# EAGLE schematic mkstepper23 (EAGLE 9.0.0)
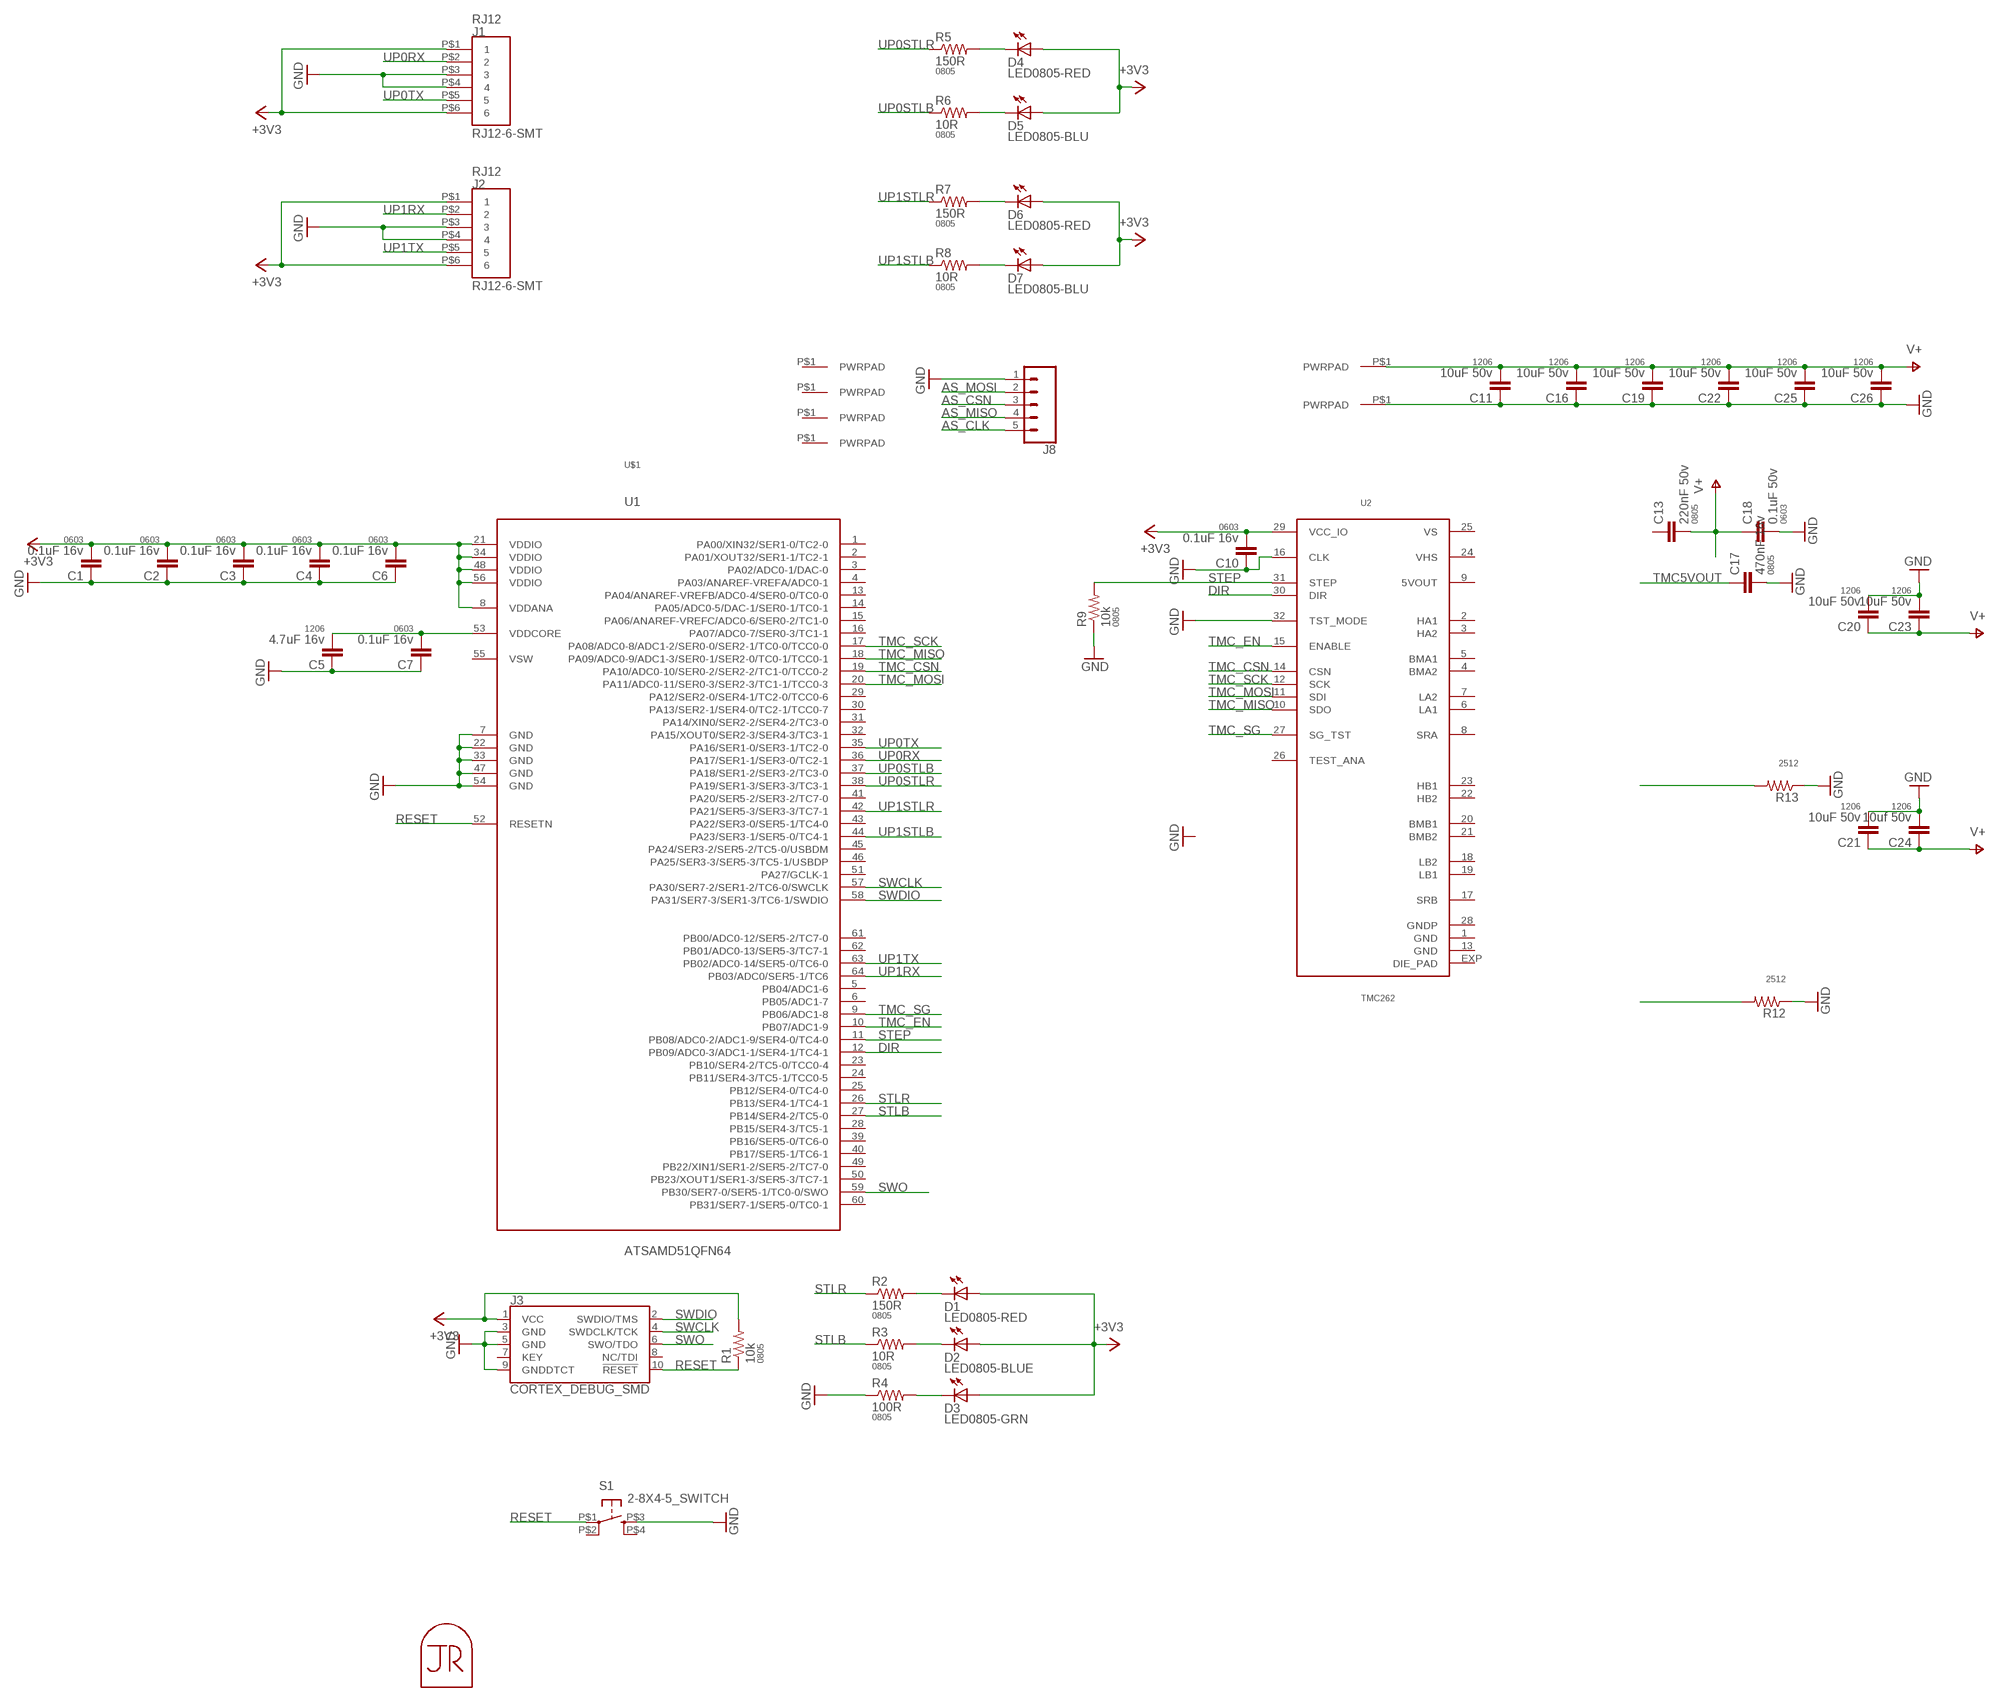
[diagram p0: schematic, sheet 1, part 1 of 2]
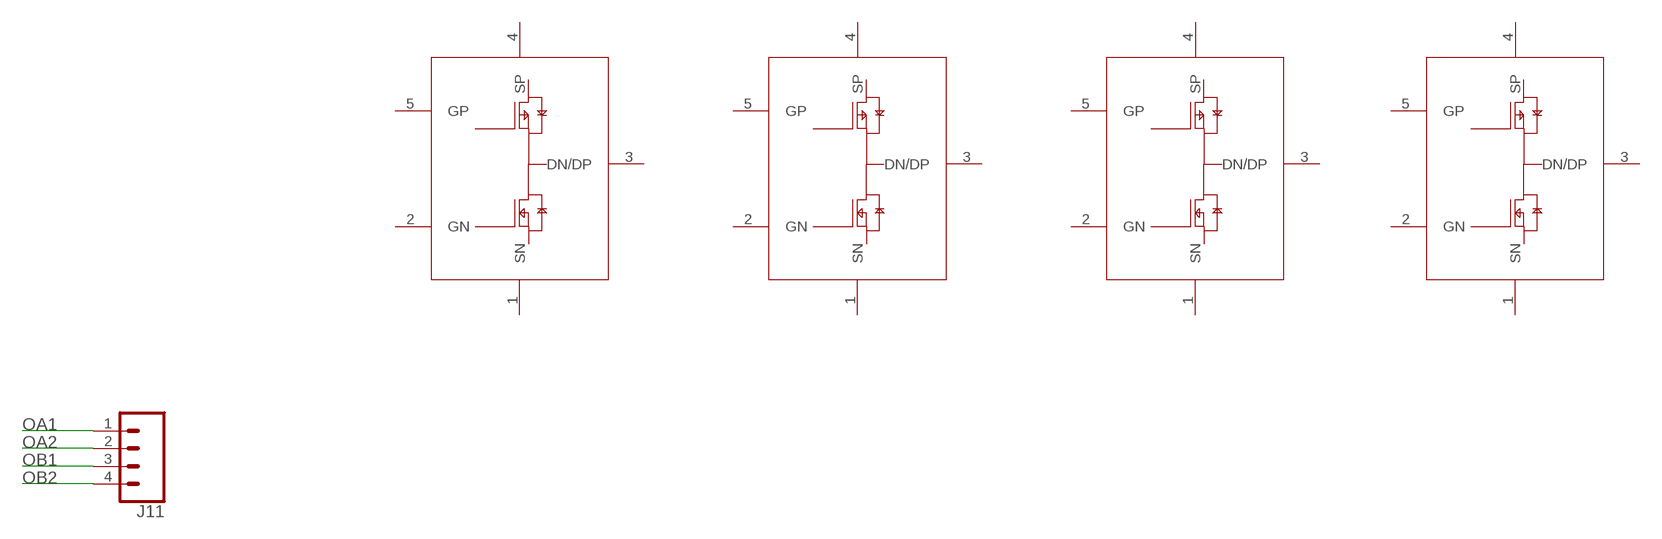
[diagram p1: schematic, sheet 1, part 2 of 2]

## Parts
C1  0.1uF 16v  CAP0603-CAP  [0603-CAP]
C2  0.1uF 16v  CAP0603-CAP  [0603-CAP]
C3  0.1uF 16v  CAP0603-CAP  [0603-CAP]
C4  0.1uF 16v  CAP0603-CAP  [0603-CAP]
C5  4.7uF 16v  CAP1206  [1206]
C6  0.1uF 16v  CAP0603-CAP  [0603-CAP]
C7  0.1uF 16v  CAP0603-CAP  [0603-CAP]
C10  0.1uF 16v  CAP0603-CAP  [0603-CAP]
C11  10uF 50v  CAP1206  [1206]
C13  220nF 50v  CAP0805  [0805]
C16  10uF 50v  CAP1206  [1206]
C17  470nF 16v  CAP0805  [0805]
C18  0.1uF 50v  CAP0603-CAP  [0603-CAP]
C19  10uF 50v  CAP1206  [1206]
C20  10uF 50v  CAP1206  [1206]
C21  10uF 50v  CAP1206  [1206]
C22  10uF 50v  CAP1206  [1206]
C23  10uF 50v  CAP1206  [1206]
C24  10uf 50v  CAP1206  [1206]
C25  10uF 50v  CAP1206  [1206]
C26  10uF 50v  CAP1206  [1206]
D1  LED0805-RED  LED0805  [LED0805]
D2  LED0805-BLUE  LED0805  [LED0805]
D3  LED0805-GRN  LED0805  [LED0805]
D4  LED0805-RED  LED0805  [LED0805]
D5  LED0805-BLU  LED0805  [LED0805]
D6  LED0805-RED  LED0805  [LED0805]
D7  LED0805-BLU  LED0805  [LED0805]
J1  RJ12-6-SMT  [RJ12-6-SMT]
J2  RJ12-6-SMT  [RJ12-6-SMT]
J3  CORTEX_DEBUG_SMD  [SAMTECH_FTSH-105-01]
J4  PWRPADM3  [PWRPAD_3-25MM]
J5  PWRPADM3  [PWRPAD_3-25MM]
J6  PWRPADM3  [PWRPAD_3-25MM]
J7  PWRPADM3  [PWRPAD_3-25MM]
J8  CONN_05NO_SILK  [1X05_NO_SILK]
J9  PWRPAD  [PWRPAD_M3-PEM-MOUNT]
J10  PWRPAD  [PWRPAD_M3-PEM-MOUNT]
J11  CONN_04LONGPADS  [1X04_LONGPADS]
MP1  JRTOMBSTONE  [JRTOMBSTONE]
Q1  PNPAIR-FDD8424H  [DPAK-5]
Q2  PNPAIR-FDD8424H  [DPAK-5]
Q3  PNPAIR-FDD8424H  [DPAK-5]
Q4  PNPAIR-FDD8424H  [DPAK-5]
R1  10k  RESISTOR0805-RES  [0805]
R2  150R  RESISTOR0805-RES  [0805]
R3  10R  RESISTOR0805-RES  [0805]
R4  100R  RESISTOR0805-RES  [0805]
R5  150R  RESISTOR0805-RES  [0805]
R6  10R  RESISTOR0805-RES  [0805]
R7  150R  RESISTOR0805-RES  [0805]
R8  10R  RESISTOR0805-RES  [0805]
R9  10k  RESISTOR0805-RES  [0805]
R12  RESISTOR2512  [R2512]
R13  RESISTOR2512  [R2512]
S1  2-8X4-5_SWITCH  [TACT-SWITCH-KMR6]
U1  ATSAMD51QFN64  [QFN-64-9X9MM]
U2  TMC262  [QFN32]
U$1  NEMA23  [NEMA23]

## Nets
+3V3: C1.2 C2.2 C3.2 C4.2 C6.2 C10.2 D1.1(A) D2.1(A) D3.1(A) D4.1(A) D5.1(A) D6.1(A) D7.1(A) J1.P$1 J1.P$6 J2.P$1 J2.P$6 J3.1(VCC) R1.2 U1.8(VDDANA) U1.21(VDDIO) U1.34(VDDIO) U1.48(VDDIO) U1.56(VDDIO) U2.29(VCC_IO)
AS_CLK: J8.5
AS_CSN: J8.3
AS_MISO: J8.4
AS_MOSI: J8.2
BRA: R13.2
BRB: R12.2
DIR: U1.12(PB09/ADC0-3/ADC1-1/SER4-1/TC4-1) U2.30(DIR)
GND: C1.1 C2.1 C3.1 C4.1 C5.1 C6.1 C7.1 C10.1 C11.1 C16.1 C17.2 C18.2 C19.1 C20.2 C21.2 C22.1 C23.2 C24.2 C25.1 C26.1 J1.P$3 J1.P$4 J2.P$3 J2.P$4 J3.3(GND) J3.5(GND) J3.9(GNDDTCT) J8.1 J10.P$1(PWRPAD) R4.1 R9.1 R12.1 R13.1 S1.P$3(S) U1.7(GND) U1.22(GND) U1.33(GND) U1.47(GND) U1.54(GND) U2.16(CLK) U2.32(TST_MODE)
N$1: D3.2(C) R4.2
N$5: D2.2(C) R3.2
N$6: D1.2(C) R2.2
N$7: C5.2 C7.2 U1.53(VDDCORE)
N$10: D4.2(C) R5.2
N$11: D5.2(C) R6.2
N$13: D6.2(C) R7.2
N$14: D7.2(C) R8.2
OA1: J11.1
OA2: J11.2
OB1: J11.3
OB2: J11.4
RESET: J3.10(!RESET) R1.1 S1.P$1(P) U1.52(RESETN)
STEP: R9.2 U1.11(PB08/ADC0-2/ADC1-9/SER4-0/TC4-0) U2.31(STEP)
STLB: R3.1 U1.27(PB14/SER4-2/TC5-0)
STLR: R2.1 U1.26(PB13/SER4-1/TC4-1)
SWCLK: J3.4(SWDCLK/TCK) U1.57(PA30/SER7-2/SER1-2/TC6-0/SWCLK)
SWDIO: J3.2(SWDIO/TMS) U1.58(PA31/SER7-3/SER1-3/TC6-1/SWDIO)
SWO: J3.6(SWO/TDO) U1.59(PB30/SER7-0/SER5-1/TC0-0/SWO)
TMC5VOUT: C17.1
TMC_CSN: U1.19(PA10/ADC0-10/SER0-2/SER2-2/TC1-0/TCC0-2) U2.14(CSN)
TMC_EN: U1.10(PB07/ADC1-9) U2.15(ENABLE)
TMC_MISO: U1.18(PA09/ADC0-9/ADC1-3/SER0-1/SER2-0/TC0-1/TCC0-1) U2.10(SDO)
TMC_MOSI: U1.20(PA11/ADC0-11/SER0-3/SER2-3/TC1-1/TCC0-3) U2.11(SDI)
TMC_SCK: U1.17(PA08/ADC0-8/ADC1-2/SER0-0/SER2-1/TC0-0/TCC0-0) U2.12(SCK)
TMC_SG: U1.9(PB06/ADC1-8) U2.27(SG_TST)
UP0RX: J1.P$2 U1.36(PA17/SER1-1/SER3-0/TC2-1)
UP0STLB: R6.1 U1.37(PA18/SER1-2/SER3-2/TC3-0)
UP0STLR: R5.1 U1.38(PA19/SER1-3/SER3-3/TC3-1)
UP0TX: J1.P$5 U1.35(PA16/SER1-0/SER3-1/TC2-0)
UP1RX: J2.P$2 U1.64(PB03/ADC0/SER5-1/TC6)
UP1STLB: R8.1 U1.44(PA23/SER3-1/SER5-0/TC4-1)
UP1STLR: R7.1 U1.42(PA21/SER5-3/SER3-3/TC7-1)
UP1TX: J2.P$5 U1.63(PB02/ADC0-14/SER5-0/TC6-0)
V+: C11.2 C13.2 C16.2 C18.1 C19.2 C20.1 C21.1 C22.2 C23.1 C24.1 C25.2 C26.2 J9.P$1(PWRPAD)
Unconnected: C13.1 J3.7(KEY) J3.8(NC/TDI) J4.P$1(PWRPAD) J5.P$1(PWRPAD) J6.P$1(PWRPAD) J7.P$1(PWRPAD) Q1.1(SN) Q1.2(GN) Q1.3(DN/DP) Q1.4(SP) Q1.5(GP) Q2.1(SN) Q2.2(GN) Q2.3(DN/DP) Q2.4(SP) Q2.5(GP) Q3.1(SN) Q3.2(GN) Q3.3(DN/DP) Q3.4(SP) Q3.5(GP) Q4.1(SN) Q4.2(GN) Q4.3(DN/DP) Q4.4(SP) Q4.5(GP) S1.P$2(P1) S1.P$4(S1) U1.1(PA00/XIN32/SER1-0/TC2-0) U1.2(PA01/XOUT32/SER1-1/TC2-1) U1.3(PA02/ADC0-1/DAC-0) U1.4(PA03/ANAREF-VREFA/ADC0-1) U1.5(PB04/ADC1-6) U1.6(PB05/ADC1-7) U1.13(PA04/ANAREF-VREFB/ADC0-4/SER0-0/TC0-0) U1.14(PA05/ADC0-5/DAC-1/SER0-1/TC0-1) U1.15(PA06/ANAREF-VREFC/ADC0-6/SER0-2/TC1-0) U1.16(PA07/ADC0-7/SER0-3/TC1-1) U1.23(PB10/SER4-2/TC5-0/TCC0-4) U1.24(PB11/SER4-3/TC5-1/TCC0-5) U1.25(PB12/SER4-0/TC4-0) U1.28(PB15/SER4-3/TC5-1) U1.29(PA12/SER2-0/SER4-1/TC2-0/TCC0-6) U1.30(PA13/SER2-1/SER4-0/TC2-1/TCC0-7) U1.31(PA14/XIN0/SER2-2/SER4-2/TC3-0) U1.32(PA15/XOUT0/SER2-3/SER4-3/TC3-1) U1.39(PB16/SER5-0/TC6-0) U1.40(PB17/SER5-1/TC6-1) U1.41(PA20/SER5-2/SER3-2/TC7-0) U1.43(PA22/SER3-0/SER5-1/TC4-0) U1.45(PA24/SER3-2/SER5-2/TC5-0/USBDM) U1.46(PA25/SER3-3/SER5-3/TC5-1/USBDP) U1.49(PB22/XIN1/SER1-2/SER5-2/TC7-0) U1.50(PB23/XOUT1/SER1-3/SER5-3/TC7-1) U1.51(PA27/GCLK-1) U1.55(VSW) U1.60(PB31/SER7-1/SER5-0/TC0-1) U1.61(PB00/ADC0-12/SER5-2/TC7-0) U1.62(PB01/ADC0-13/SER5-3/TC7-1) U2.1(GND) U2.2(HA1) U2.3(HA2) U2.4(BMA2) U2.5(BMA1) U2.6(LA1) U2.7(LA2) U2.8(SRA) U2.9(5VOUT) U2.13(GND) U2.17(SRB) U2.18(LB2) U2.19(LB1) U2.20(BMB1) U2.21(BMB2) U2.22(HB2) U2.23(HB1) U2.24(VHS) U2.25(VS) U2.26(TEST_ANA) U2.28(GNDP) U2.EXP(DIE_PAD)

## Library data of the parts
C1-C4 C6 C7 C10 C18 = borkedlabs-passives:CAP: Capacitor; PACKAGE: 0603
C5 C11 C16 C19-C26 = borkedlabs-passives:CAP: Capacitor; PACKAGE: 1206
C13 C17 = borkedlabs-passives:CAP: Capacitor; PACKAGE: 0805
D1-D7 = lights:LED: LED
J1 J2 = connector:RJ12-6-SMT
J3 = SparkFun-Connectors:CORTEX_DEBUG: Cortex Debug Connector - 10 pin Supports JTAG debug, Serial Wire debug, and Serial Wire Viewer. PTH and SMD connector options available. General Connector Information Products: PTH Connector -via Digi-Key SparkFun PSoc SparkFun T
J4-J7 J9 J10 = power:PWRPAD
J8 = SparkFun-Connectors:CONN_05: Multi connection point. Often used as Generic Header-pin footprint for 0.1 inch spaced/style header connections On any of the 0.1 inch spaced packages, you can populate with these: Break Away Headers - Straight (PRT-00116) Break Away Male Headers - Right Angle (PRT-00553) Female Headers (PRT-00115)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
J11 = SparkFun-Connectors:CONN_04: Multi connection point. Often used as Generic Header-pin footprint for 0.1 inch spaced/style header connections On any of the 0.1 inch spaced packages, you can populate with these: Break Away Headers - Straight (PRT-00116) Break Away Male Headers - Right Angle (PRT-00553) Female Headers (PRT-00115)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; PROD_ID: CONN-09696
MP1 = connector:JRTOMBSTONE
Q1-Q4 = power:PNPAIR-FDD8424H
R1-R9 = borkedlabs-passives:RESISTOR: Resistor; PACKAGE: 0805
R12 R13 = borkedlabs-passives:RESISTOR: Resistor; PACKAGE: 2512
S1 = fab:2-8X4-5_SWITCH
U1 = atsam:ATSAMD51
U2 = power:TMC262
U$1 = motors:NEMA23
